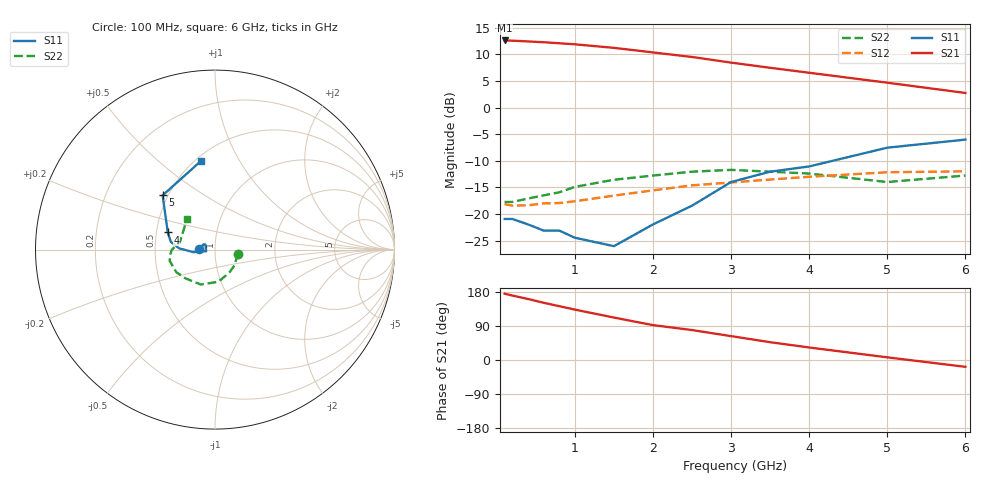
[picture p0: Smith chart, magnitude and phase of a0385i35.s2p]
!  MSA-0385 S AND NOISE PARAMETERS
!  Id=35mA  LAST UPDATED 07-22-92
# ghz s ma r 50
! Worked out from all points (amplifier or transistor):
!   14 points, 100 MHz to 6 GHz, reference 50 ohm
!   highest |S21| = 12.6 dB at 100 MHz (marker M1)
!   |S21| within 3 dB of that: start of sweep to 2.44 GHz
!   unconditionally stable (mu >= 1): start of sweep to end of sweep
!   at 400 MHz: K = 1.21, MAG = 12.6 dB, |S12| = -18.3 dB
!   at 2 GHz: K = 1.12, MAG = 10.8 dB, |S12| = -15.5 dB
!   at 6 GHz: K = 1.23, MAG = 4.5 dB, |S12| = -12.0 dB
!   lowest NFmin = 5.60 dB at 100 MHz
!   S11 on the Smith chart (normalised r, x): 100 MHz: 0.83, +0.01; 4 GHz: 0.57, +0.12; 5 GHz: 0.47, +0.34; 6 GHz: 0.53, +0.70
0.1  0.09 178.0  4.26 175.0  0.124 2.0  0.13 -10.0
0.2  0.09 171.0  4.24 170.0  0.12 3.0  0.13 -20.0
0.4  0.08 166.0  4.17 161.0  0.121 6.0  0.14 -41.0
0.6  0.07 160.0  4.1 151.0  0.126 8.0  0.15 -57.0
0.8  0.07 155.0  4.01 142.0  0.127 12.0  0.16 -71.0
1  0.06 152.0  3.92 133.0  0.132 12.0  0.18 -84.0
1.5  0.05 -169.0  3.63 112.0  0.149 18.0  0.21 -112.0
2  0.08 -174.0  3.29 92.0  0.167 19.0  0.23 -136.0
2.5  0.12 -173.0  2.98 79.0  0.186 22.0  0.25 -150.0
3  0.2 178.0  2.64 63.0  0.198 20.0  0.26 -166.0
3.5  0.25 170.0  2.36 47.0  0.211 17.0  0.25 -174.0
4  0.28 160.0  2.12 33.0  0.224 13.0  0.24 -180.0
5  0.42 134.0  1.71 7.0  0.247 4.0  0.2 168.0
6  0.5 99.0  1.37 -18.0  0.252 -7.0  0.23 133.0
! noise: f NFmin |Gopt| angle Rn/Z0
0.1  5.6  0.05  2  0.84
0.5  5.8  0.04  11  0.84
1  6  0.03  11  0.83
2  6.5  0.01  -178  0.8
